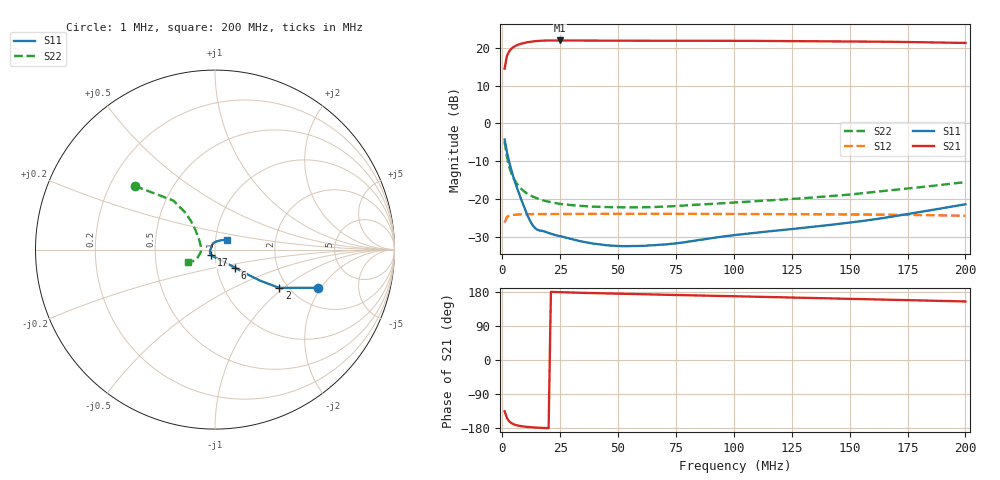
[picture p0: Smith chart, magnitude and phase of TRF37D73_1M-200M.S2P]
!Agilent Technologies,E5071B,JP1KK00322,A.09.10
!Date: Mon Jul 07 16:55:38 2014
!Data & Calibration Information:
!Freq		S11:SOLT2(ON)  S21:SOLT2(ON)  S12:SOLT2(ON)  S22:SOLT2(ON)
# Hz S dB R 50
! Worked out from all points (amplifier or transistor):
!   200 points, 1 MHz to 200 MHz, reference 50 ohm
!   highest |S21| = 21.9 dB at 25 MHz (marker M1)
!   |S21| within 3 dB of that: 2.883 MHz to end of sweep
!   unconditionally stable (mu >= 1): start of sweep to end of sweep
!   at 34 MHz: K = 1.03, MAG = 21.9 dB, |S12| = -23.9 dB
!   at 101 MHz: K = 1.03, MAG = 21.9 dB, |S12| = -24.0 dB
!   at 200 MHz: K = 1.05, MAG = 21.5 dB, |S12| = -24.5 dB
!   S11 on the Smith chart (normalised r, x): 1 MHz: 2.75, -1.87; 2 MHz: 1.81, -0.93; 6 MHz: 1.22, -0.25; 17 MHz: 0.96, -0.06; 200 MHz: 1.14, +0.12
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1000000  -4.28 -20.4  14.46 -135.3  -26.24 40.5  -4.86 141.6
2000000  -7.60 -30.8  17.82 -153.5  -24.78 22.9  -8.91 130.3
3000000  -10.28 -34.5  19.06 -162.0  -24.42 15.9  -11.54 128.8
4000000  -12.57 -37.0  19.76 -166.8  -24.27 12.2  -13.36 129.9
5000000  -14.60 -39.3  20.23 -169.8  -24.19 9.8  -14.70 131.7
6000000  -16.47 -42.1  20.57 -171.8  -24.14 8.2  -15.73 133.8
7000000  -18.21 -45.3  20.82 -173.3  -24.10 7.1  -16.55 135.9
8000000  -19.87 -49.2  21.03 -174.5  -24.08 6.2  -17.22 137.8
1.1e7  -24.54 -68.6  21.46 -176.7  -24.03 4.3  -18.66 143.3
1.4e7  -27.61 -95.9  21.71 -178.1  -24.00 3.2  -19.60 148.0
1.7e7  -28.42 -123.0  21.85 -179.2  -23.98 2.4  -20.27 152.0
2e7  -28.99 -135.6  21.90 -180.0  -23.96 1.6  -20.75 155.5
2.5e7  -29.84 -150.2  21.91 178.9  -23.94 0.8  -21.30 160.5
3.5e7  -31.34 -171.2  21.88 177.2  -23.93 -0.6  -21.89 168.5
4.9e7  -32.43 165.0  21.85 175.1  -23.92 -2.0  -22.20 177.1
6.8e7  -32.11 140.6  21.84 172.5  -23.92 -3.7  -22.09 -173.2
1.01e8  -29.52 114.5  21.82 168.1  -23.97 -6.4  -20.92 -162.7
1.34e8  -27.40 87.4  21.74 163.7  -24.04 -8.9  -19.62 -156.2
1.51e8  -26.18 73.1  21.67 161.4  -24.08 -10.3  -18.78 -153.3
1.67e8  -24.80 61.5  21.57 159.1  -24.16 -11.9  -17.77 -152.2
1.88e8  -22.67 46.7  21.39 156.1  -24.32 -13.7  -16.39 -153.0
2e8  -21.41 37.7  21.26 154.5  -24.46 -14.8  -15.54 -154.7
